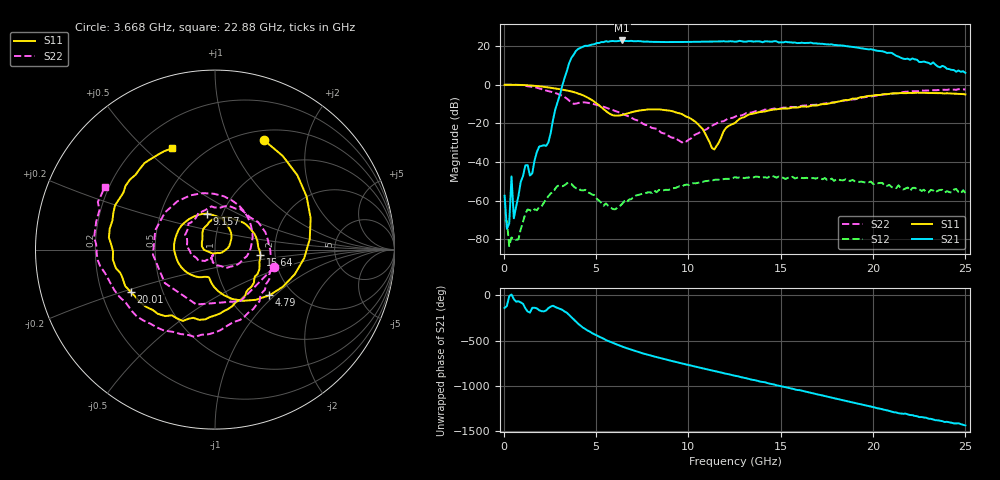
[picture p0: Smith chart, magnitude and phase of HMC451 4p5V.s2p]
!Hittite Microwave Corporation
!20 Alpha Road
!Chelmsford, MA 01824
!Tel: 978-250-3343
!Fax: 978-250-3373
!Device: HMC451, 5-20 GHz, Driver Amplifier Die
!Misc: Vcc = 4.5V, room. Die measured in housing that includes two K connectors, not de-embedded.
# MHZ S MA R 50
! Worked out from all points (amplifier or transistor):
!   201 points, 50 MHz to 25 GHz, reference 50 ohm
!   highest |S21| = 22.9 dB at 6.412 GHz (marker M1)
!   |S21| within 3 dB of that: 4.349 GHz to 18.6 GHz (14.26 GHz wide, 124 % of centre)
!   unconditionally stable (mu >= 1): start of sweep to end of sweep
!   at 4.167 GHz: K = 18.16, MAG = 21.2 dB, |S12| = -54.6 dB
!   at 12.53 GHz: K = 9.30, MAG = 22.4 dB, |S12| = -47.9 dB
!   at 25 GHz: K = 46.84, MAG = 11.4 dB, |S12| = -56.0 dB
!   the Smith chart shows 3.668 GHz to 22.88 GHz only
!   S11 on the Smith chart (normalised r, x): 3.668 GHz: 0.61, +1.35; 4.79 GHz: 1.53, -0.93; 9.157 GHz: 0.85, +0.35; 15.64 GHz: 1.67, -0.11; 20.01 GHz: 0.33, -0.21; 22.88 GHz: 0.34, +0.61
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50  0.993 -3.7  0.001329 -140.9  0.0003071 -129.0  0.994 -4.1
3168.75  0.746 112.2  0.925 -160.6  0.002343 95.4  0.518 97.4
3667.75  0.669 66.2  4.966 116.8  0.002693 55.1  0.343 -16.8
3917.25  0.618 42.0  7.525 68.9  0.002089 30.7  0.323 -108.7
4291.5  0.531 6.2  9.653 2.9  0.001824 19.8  0.35 162.0
4790.5  0.396 -40.0  10.97 -58.3  0.00143 7.7  0.322 102.2
5414.25  0.232 -85.7  12.67 -119.8  0.0007342 1.4  0.267 51.9
5913.25  0.162 -101.1  13.54 -165.7  0.000601 28.2  0.221 18.3
6412.25  0.164 -112.2  13.98 154.8  0.0008176 42.7  0.181 -11.8
7285.5  0.212 -152.7  13.46 95.4  0.001402 41.7  0.118 -59.8
8408.25  0.23 144.5  12.79 31.1  0.001888 27.2  0.065 -101.4
9156.75  0.205 102.3  12.7 -7.0  0.002076 21.6  0.042 -122.4
10778.5  0.071 6.0  13 -85.2  0.003052 1.5  0.063 -116.9
12525  0.102 133.2  12.93 -167.1  0.004041 -32.3  0.148 177.8
14271.5  0.21 48.4  13.21 112.8  0.003853 -68.4  0.223 110.4
15643.75  0.255 -6.8  12.32 49.8  0.004128 -90.7  0.265 53.9
16766.5  0.29 -45.9  11.74 -1.7  0.003824 -112.7  0.3 9.9
18388.25  0.392 -97.8  10.26 -76.9  0.003339 -143.5  0.383 -52.4
20010  0.525 -153.2  8.035 -151.6  0.002667 -176.0  0.508 -112.2
20883.25  0.578 177.5  6.73 166.1  0.002538 164.8  0.576 -143.4
22879.25  0.613 113.2  3.804 90.8  0.001659 142.5  0.707 150.5
25000  0.559 49.6  2.019 6.5  0.001577 111.5  0.75 85.4
